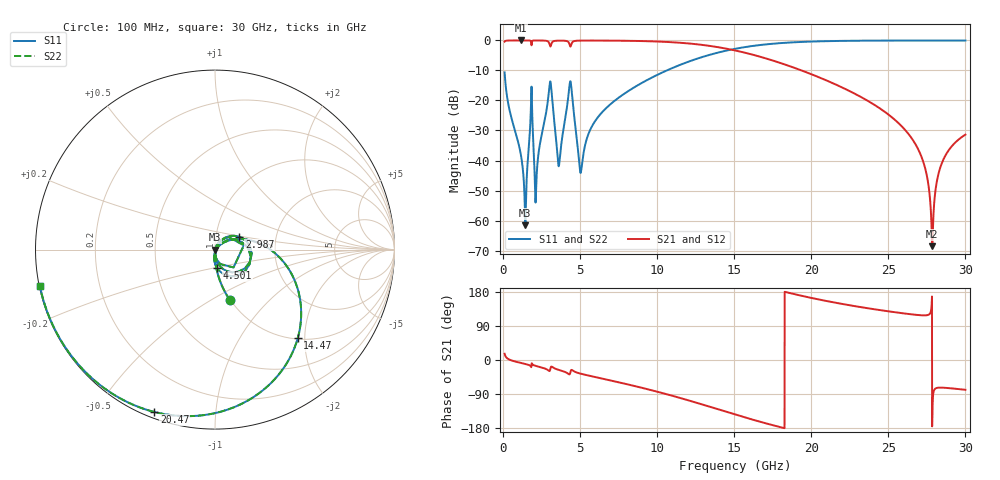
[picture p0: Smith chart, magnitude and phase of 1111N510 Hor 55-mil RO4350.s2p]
# GHz S MA R 50
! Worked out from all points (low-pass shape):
!   3201 points, 100 MHz to 30 GHz, reference 50 ohm
!   highest |S21| = -0.01 dB at 1.147 GHz (marker M1); lowest = -68.5 dB at 27.85 GHz (marker M2)
!   |S21| within 3 dB of the highest: start of sweep to 14.75 GHz
!   lowest |S11| = -61.6 dB at 1.446 GHz (marker M3), VSWR 1.00, Z = 50.1 - j0.0031 ohm
!   |S11| at or under -10 dB: start of sweep to 10.62 GHz
!   |S22| runs from -61.6 to 0.0 dB; largest |S21 - S12| = 0
!   S11 on the Smith chart (normalised r, x): 100 MHz: 0.99, -0.61; 2.987 GHz: 1.30, +0.19; 4.501 GHz: 1.00, -0.21; 14.47 GHz: 1.02, -1.85; 20.47 GHz: 0.03, -0.69; 30 GHz: 0.00, -0.10
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0.1  0.2942 -73.6  0.9555 16.4  0.9555 16.4  0.2942 -73.6
1.1465  0.01282 -95.0  0.9992 -7.6  0.9992 -7.6  0.01282 -95.0
1.4455  0.0008337 -2.1  0.999 -10.6  0.999 -10.6  0.0008337 -2.1
1.791219  0.0584 58.4  0.9828 -16.3  0.9828 -16.3  0.0584 58.4
2.164969  0.004761 51.5  0.9979 -16.0  0.9979 -16.0  0.004761 51.5
2.987219  0.1533 27.8  0.9076 -29.0  0.9076 -29.0  0.1533 27.8
3.155406  0.1301 -63.4  0.9048 -17.5  0.9048 -17.5  0.1301 -63.4
3.622594  0.008111 -11.4  0.9917 -26.3  0.9917 -26.3  0.008111 -11.4
4.286  0.1556 15.1  0.8981 -37.9  0.8981 -37.9  0.1556 15.1
4.500906  0.104 -83.3  0.9376 -27.3  0.9376 -27.3  0.104 -83.3
5.089563  0.007416 4.5  0.9938 -36.6  0.9938 -36.6  0.007416 4.5
6.294906  0.05831 39.3  0.9947 -47.8  0.9947 -47.8  0.05831 39.3
10.06978  0.2717 5.0  0.958 -84.3  0.958 -84.3  0.2717 5.0
14.47069  0.6751 -46.9  0.7309 -136.5  0.7309 -136.5  0.6751 -46.9
15.05  0.7247 -54.1  0.6818 -143.7  0.6818 -143.7  0.7247 -54.1
20.03956  0.9586 -106.9  0.2715 163.5  0.2715 163.5  0.9586 -106.9
20.46937  0.9658 -110.5  0.2451 159.9  0.2451 159.9  0.9658 -110.5
25.01978  0.9952 -142.3  0.05791 128.3  0.05791 128.3  0.9952 -142.3
27.06606  0.9969 -153.7  0.01304 118.2  0.01304 118.2  0.9969 -153.7
27.85094  0.997 -157.8  0.0003742 -153.6  0.0003742 -153.6  0.997 -157.8
28.49566  0.9969 -161.0  0.009359 -73.0  0.009359 -73.0  0.9969 -161.0
30  0.9966 -168.1  0.02697 -78.6  0.02697 -78.6  0.9966 -168.1
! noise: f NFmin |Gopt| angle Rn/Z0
0.1  0.0006582  0.7323  1.597  0.0004904
3.417  0.02833  0.784  24.74  0.02572
6.743  0.01897  0.4878  46.27  0.005482
10.06  0.02535  0.4649  63.44  0.006076
13.39  0.03685  0.5281  78.88  0.008723
16.7  0.05801  0.6443  95.49  0.01475
20.03  0.105  0.7819  114.4  0.03006
23.35  0.2429  0.8996  133.7  0.08307
26.67  1.281  0.9798  151.8  0.8716
30  0.9869  0.9732  168  0.09332
